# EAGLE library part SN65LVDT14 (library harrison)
Texas Instruments SN65LVDT14 - one driver, four receivers
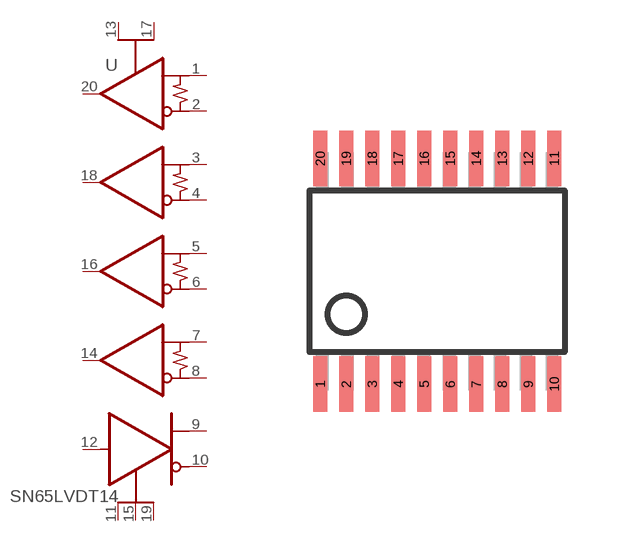
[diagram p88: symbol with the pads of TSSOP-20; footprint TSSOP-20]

Designator prefix U

## SN65LVDT14  [TSSOP-20]
1  1A  in
2  1B  in
3  2A  in
4  2B  in
5  3A  in
6  3B  in
7  4A  in
8  4B  in
9  5Y  out
10  5Z  out
11  GND1  pwr
12  5D  in
13  VCC1  pwr
14  4R  out
15  GND2  pwr
16  3R  out
17  VCC2  pwr
18  2R  out
19  GND3  pwr
20  1R  out

## Footprint TSSOP-20 (pad centres in mm)
smd 0.348 x 1.397: 1 -2.923,-2.814; 2 -2.273,-2.815; 3 -1.623,-2.815; 4 -0.973,-2.815; 5 -0.323,-2.815; 6 0.327,-2.815; 7 0.977,-2.815; 8 1.627,-2.815; 9 2.277,-2.815; 10 2.927,-2.815; 11 2.927,2.825; 12 2.277,2.825; 13 1.627,2.825; 14 0.977,2.825; 15 0.327,2.825; 16 -0.323,2.825; 17 -0.973,2.825; 18 -1.623,2.825; 19 -2.273,2.825; 20 -2.923,2.825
